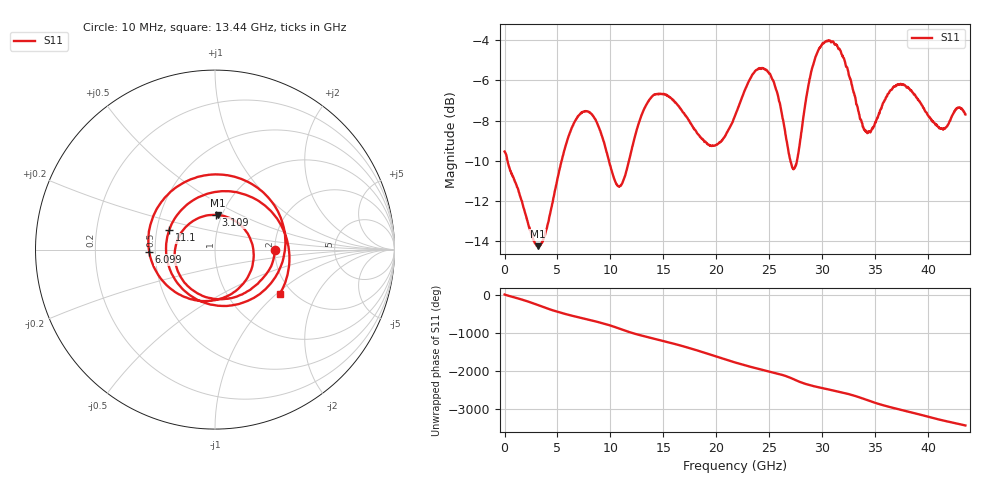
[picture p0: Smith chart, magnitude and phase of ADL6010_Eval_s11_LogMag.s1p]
!Agilent Technologies,N5224A,MY51441113,A.09.90.11
!Agilent N5224A: A.09.90.11
!Date: Wednesday, August 26, 2015 15:58:47
!Correction: S11(Full 1 Port(1))
!S1P File: Measurement: S11:
# Hz S  dB  R 50
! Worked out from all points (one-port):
!   1601 points, 10 MHz to 43.5 GHz, reference 50 ohm
!   lowest |S11| = -14.3 dB at 3.136 GHz (marker M1), VSWR 1.48, Z = 47.9 + j19.2 ohm
!   |S11| at or under -10 dB: 278 MHz to 5.392 GHz (5.114 GHz wide, 180 % of centre); 9.854 GHz to 11.75 GHz (1.901 GHz wide, 17.6 % of centre); 26.98 GHz to 27.61 GHz (624.8 MHz wide, 2.29 % of centre)
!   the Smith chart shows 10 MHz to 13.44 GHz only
!   S11 on the Smith chart (normalised r, x): 10 MHz: 2.00, -0.01; 3.109 GHz: 0.94, +0.38; 6.099 GHz: 0.46, -0.01; 11.1 GHz: 0.58, +0.14; 13.44 GHz: 1.71, -1.06
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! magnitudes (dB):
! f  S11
! 10 MHz  -9.5
! 3.109 GHz  -14.2
! 3.136 GHz  -14.3
! 3.951 GHz  -13.4
! 5.446 GHz  -9.9
! 6.099 GHz  -8.7
! 7.159 GHz  -7.7
! 8.192 GHz  -7.7
! 10.88 GHz  -11.3
! 11.1 GHz  -11.1
! 13.44 GHz  -7.2
! 16.32 GHz  -7.2
! 19.44 GHz  -9.3
! 21.75 GHz  -7.8
! 23.49 GHz  -5.6
! 24.74 GHz  -5.5
! 25.81 GHz  -6.8
! 27.19 GHz  -10.4
! 27.65 GHz  -9.9
! 28.88 GHz  -5.7
! 29.83 GHz  -4.3
! 31.24 GHz  -4.2
! 32.63 GHz  -5.9
! 34.31 GHz  -8.6
! 36.54 GHz  -6.5
! 38.06 GHz  -6.3
! 41.19 GHz  -8.4
! 43.5 GHz  -7.7
